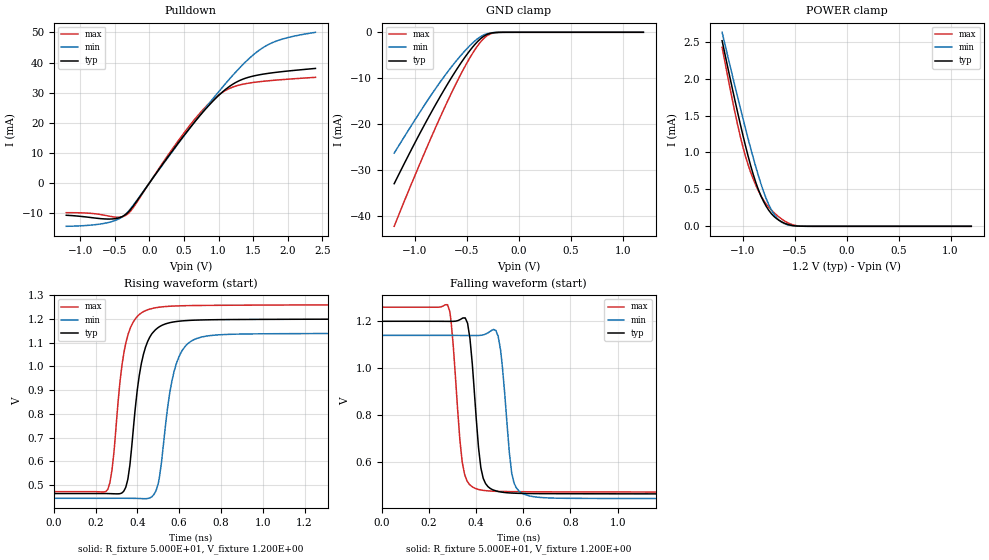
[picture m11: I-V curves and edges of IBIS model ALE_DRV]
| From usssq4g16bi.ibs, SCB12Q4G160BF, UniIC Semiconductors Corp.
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|   Model ALE_DRV
[Model] ALE_DRV
Model_type Open_sink
Polarity   Non-Inverting
Enable   Active-High
Vmeas =  6.000E-01
Rref =  5.000E+01
Vref =  1.200E+00
C_comp   6.021E-13   5.870E-13   6.180E-13
C_comp_pulldown   4.780E-13   4.385E-13   5.674E-13
C_comp_power_clamp   1.241E-13   5.058E-14   1.485E-13
[Model Spec]
Vmeas   6.000E-01   5.700E-01   6.300E-01
Vref   1.200E+00   1.140E+00   1.260E+00
Rref   5.000E+01   5.000E+01   5.000E+01
[Temperature Range]   45.000   95.000   -40.000
[Voltage Range]   1.200E+00   1.140E+00   1.260E+00
[C Comp Corner]
C_comp_pulldown   4.780E-13   4.385E-13   5.674E-13
C_comp_power_clamp   1.241E-13   1.485E-13   5.058E-14
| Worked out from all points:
|   slope of the pulldown table from 0 to 0.18 V, typ, clamps not added: 30.8 ohm
|   GND clamp passes 1 mA (typ) near -0.35 V on its own axis
|   POWER clamp passes 1 mA (typ) near -0.96 V on its own axis
|   rising waveform, R_fixture 5.000E+01, V_fixture 1.200E+00: 20-80 % time 62.4ps typ, 69.4ps min, 59ps max; typ from 0.464 V to 1.2 V
|   falling waveform, R_fixture 5.000E+01, V_fixture 1.200E+00: 20-80 % time 35.4ps typ, 35.7ps min, 35.5ps max; typ from 1.2 V to 0.465 V
[Pulldown]
|Voltage   I(typ)   I(min)   I(max)
-1.2V     -10.69mA   -14.35mA   -9.84mA
-608mV    -11.94mA   -13.18mA   -10.85mA
-423mV    -11.42mA   -11.67mA   -11.32mA
-312mV    -9.822mA   -9.629mA   -10.26mA
-238mV    -7.806mA   -7.55mA    -8.327mA
576mV     18.01mA    17.91mA    18.87mA
872mV     26.05mA    26.64mA    26.64mA
1.094V    30.95mA    32.82mA    30.64mA
1.353V    34.49mA    39.36mA    32.8mA
1.686V    36.29mA    45.54mA    33.86mA
1.945V    37.03mA    47.93mA    34.37mA
2.4V      38.03mA    50.03mA    35.08mA
[GND_clamp]
|Voltage   I(typ)   I(min)   I(max)
-1.2V     -32.89mA   -26.25mA   -42.15mA
-1.05V    -26.17mA   -20.81mA   -33.8mA
-900mV    -19.74mA   -15.53mA   -25.78mA
-775mV    -14.67mA   -11.37mA   -19.35mA
-650mV    -9.913mA   -7.565mA   -13.25mA
-550mV    -6.428mA   -4.817mA   -8.75mA
-450mV    -3.367mA   -2.432mA   -4.753mA
-375mV    -1.535mA   -1.055mA   -2.293mA
-325mV    -689.4uA   -458.9uA   -1.089mA
-250mV    -113.6uA   -79.32uA   -186uA
-175mV    -10.33uA   -8.935uA   -14.22uA
1.2V      0A         0A         0A
[POWER_clamp]
|Voltage   I(typ)   I(min)   I(max)
-1.2V     2.514mA    2.628mA    2.425mA
-1.125V   2.017mA    2.182mA    1.878mA
-1.05V    1.538mA    1.746mA    1.372mA
-1V       1.235mA    1.463mA    1.077mA
-950mV    952.5uA    1.189mA    833.5uA
-875mV    591.3uA    802uA      554.9uA
-800mV    333.7uA    467uA      351.1uA
-725mV    169.9uA    220.7uA    219uA
-650mV    79.46uA    80.36uA    123.7uA
-550mV    18.75uA    13.3uA     35.96uA
-425mV    915.2nA    774.2nA    1.575uA
1.2V      0A         0A         9.82nA
[Ramp]
| variable   typ   min   max
dV/dt_r   4.410E-01/6.483E-11   4.168E-01/7.198E-11   4.722E-01/6.224E-11
dV/dt_f   4.412E-01/3.767E-11   4.172E-01/3.989E-11   4.725E-01/3.598E-11
R_load = 5.000E+01
[Rising Waveform]
R_fixture= 5.000E+01
V_fixture= 1.200E+00
V_fixture_min= 1.140E+00
V_fixture_max= 1.260E+00
|time   V(typ)   V(min)   V(max)
0s        464.4mV    444.4mV    472.4mV
258ps     464.2mV    444.4mV    481.5mV
279ps     463.7mV    444.5mV    568.4mV
334ps     473.3mV    444.5mV    1.048V
355ps     528.3mV    444.4mV    1.133V
439ps     1.081V     442.8mV    1.234V
499ps     1.163V     503.5mV    1.248V
585ps     1.188V     1.007V     1.254V
666ps     1.194V     1.11V      1.256V
2ns       1.199V     1.139V     1.259V
[Falling Waveform]
R_fixture= 5.000E+01
V_fixture= 1.200E+00
V_fixture_min= 1.140E+00
V_fixture_max= 1.260E+00
|time   V(typ)   V(min)   V(max)
0s        1.2V       1.14V      1.26V
279ps     1.2V       1.14V      1.27V
341ps     1.212V     1.14V      602.7mV
364ps     1.191V     1.14V      516.8mV
401ps     781.1mV    1.139V     487mV
430ps     532.3mV    1.142V     480.3mV
493ps     475.7mV    1.137V     475.8mV
551ps     468.7mV    553.9mV    474.8mV
605ps     467mV      463.3mV    474.3mV
2ns       464.7mV    444.7mV    472.6mV
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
